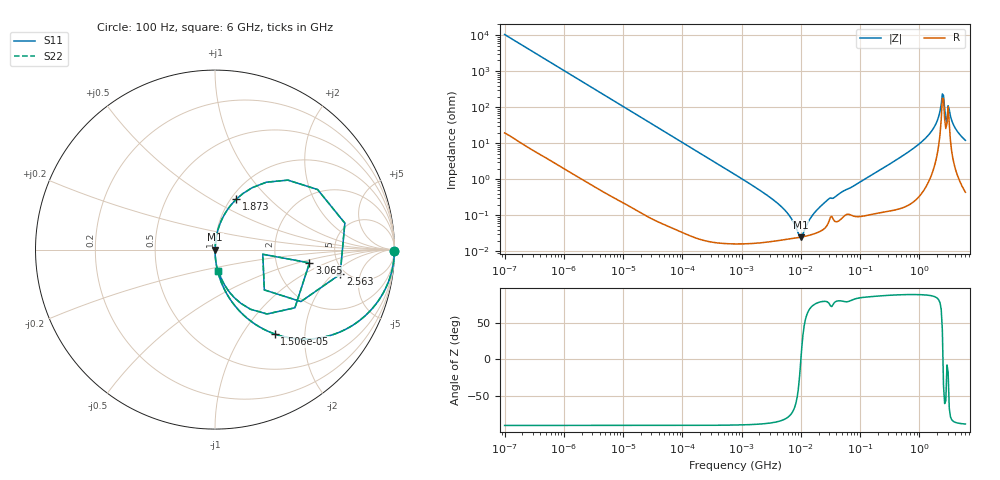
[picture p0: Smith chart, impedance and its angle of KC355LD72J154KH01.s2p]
!Murata Part Number: KC355LD72J154KH01
!These Parameters are Measured in Series Mode Connection
!Data Generated on Jun 19, 2026
!  o--ll--o
!Port1  Port2
!  o------o
!Operation Temp=25[degC], DC Bias Voltage=0[V]
!Freq. Start=100[Hz] Stop=6[GHz] 401[Steps]
# Hz S RI R 50
!Freq.(Hz) S11(Real) S11(Imag) S21(Real) S21(Imag) S12(Real) S12(Imag) S22(Real) S22(Imag)
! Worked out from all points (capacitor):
!   401 points, 100 Hz to 6 GHz, reference 50 ohm
!   read as one part in series: C = 151 nF near 109 Hz
!   lowest |Z| = 25 mohm at 9.942 MHz (marker M1)
!   series resonance near 10.03 MHz, so ESL is about 1.7 nH
!   S11 on the Smith chart (normalised r, x): 100 Hz: open; 15.06 kHz: 1.00, -1.41; 1.873 GHz: 1.06, +0.65; 2.563 GHz: 4.48, -2.49; 3.065 GHz: 3.12, -0.65; 6 GHz: 1.01, -0.24
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100  0.9999 -0.00949  0.000108 0.00949  0.000108 0.00949  0.9999 -0.00949
2008  0.9649 -0.1831  0.0351 0.1831  0.0351 0.1831  0.9649 -0.1831
5143  0.8087 -0.3924  0.1913 0.3924  0.1913 0.3924  0.8087 -0.3924
15062  0.3317 -0.4698  0.6683 0.4698  0.6683 0.4698  0.3317 -0.4698
40335  0.0653 -0.2459  0.9347 0.2459  0.9347 0.2459  0.0653 -0.2459
135116  0.00642 -0.0782  0.9936 0.0782  0.9936 0.0782  0.00642 -0.0782
774597  0.000348 -0.0136  0.9997 0.0136  0.9997 0.0136  0.000348 -0.0136
4643984  0.000209 -0.00177  0.9998 0.00177  0.9998 0.00177  0.000209 -0.00177
6644369  0.000225 -0.000882  0.9998 0.000882  0.9998 0.000882  0.000225 -0.000882
9941735  0.00025 -1.75e-05  0.9998 1.75e-05  0.9998 1.75e-05  0.00025 -1.75e-05
1.555665e7  0.000298 0.00094  0.9997 -0.00094  0.9997 -0.00094  0.000298 0.00094
2.911731e7  0.000626 0.00274  0.9994 -0.00274  0.9994 -0.00274  0.000626 0.00274
3.124326e8  0.00201 0.0263  0.998 -0.0263  0.998 -0.0263  0.00201 0.0263
1.046602e9  0.0142 0.1018  0.9858 -0.1018  0.9858 -0.1018  0.0142 0.1018
1.873145e9  0.1182 0.2803  0.8818 -0.2803  0.8818 -0.2803  0.1182 0.2803
2.240541e9  0.406 0.387  0.594 -0.387  0.594 -0.387  0.406 0.387
2.450438e9  0.7234 0.1475  0.2766 -0.1475  0.2766 -0.1475  0.7234 0.1475
2.562649e9  0.6976 -0.1372  0.3024 0.1372  0.3024 0.1372  0.6976 -0.1372
3.065283e9  0.5265 -0.0741  0.4735 0.0741  0.4735 0.0741  0.5265 -0.0741
3.352442e9  0.2898 -0.3587  0.7102 0.3587  0.7102 0.3587  0.2898 -0.3587
4.009986e9  0.0848 -0.2422  0.9152 0.2422  0.9152 0.2422  0.0848 -0.2422
6e9  0.0187 -0.1187  0.9813 0.1187  0.9813 0.1187  0.0187 -0.1187
